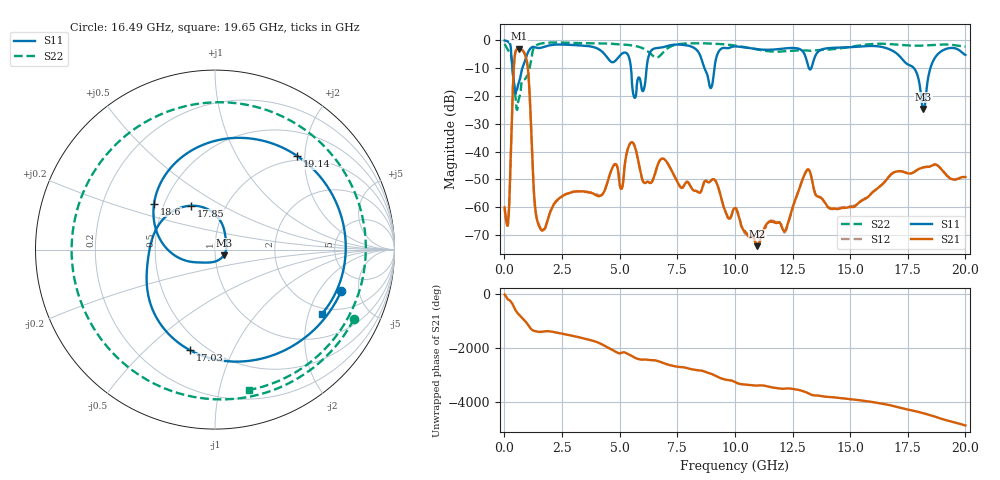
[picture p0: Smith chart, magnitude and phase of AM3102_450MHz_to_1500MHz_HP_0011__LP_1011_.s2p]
!Agilent Technologies,E8364B,MY43040894,A.07.50.67
!Agilent E8364B: A.07.50.67
!Date: Thursday, January 11, 2018 05:33:03
!Correction: S11(Full 2 Port(1,2))
!S21(Full 2 Port(1,2))
!S12(Full 2 Port(1,2))
!S22(Full 2 Port(1,2))
!S2P File: Measurements: S11, S21, S12, S22:
# Hz S  dB  R 50
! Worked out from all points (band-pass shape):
!   1601 points, 10 MHz to 20 GHz, reference 50 ohm
!   highest |S21| = -3.02 dB at 622.2 MHz (marker M1); lowest = -74.0 dB at 10.98 GHz (marker M2)
!   |S21| within 3 dB of the highest: 445.7 MHz to 929.8 MHz (484.1 MHz wide, 70.4 % of centre)
!   lowest |S11| = -24.7 dB at 18.18 GHz (marker M3), VSWR 1.12, Z = 55.1 - j3.4 ohm
!   |S11| at or under -10 dB: 5.492 GHz to 6.169 GHz (676.9 MHz wide, 11.6 % of centre); 8.68 GHz to 9.112 GHz (431.9 MHz wide, 4.86 % of centre); 17.77 GHz to 18.48 GHz (714.4 MHz wide, 3.94 % of centre)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
!   |S22| runs from -25.0 to -0.8 dB; largest |S21 - S12| = 0.0065
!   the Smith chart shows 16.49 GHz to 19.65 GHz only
!   S11 on the Smith chart (normalised r, x): 16.49 GHz: 3.21, -3.27; 17.03 GHz: 0.41, -0.69; 17.85 GHz: 0.69, +0.36; 18.6 GHz: 0.44, +0.28; 19.14 GHz: 0.91, +1.84; 19.65 GHz: 1.76, -2.44
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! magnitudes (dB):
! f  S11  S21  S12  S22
! 10 MHz  -0.1  -60.1  -60.4  -1.3
! 172.4 MHz  -0.6  -64.2  -64.4  -3.7
! 422.3 MHz  -15.5  -8.2  -8.2  -16.5
! 622.2 MHz  -15.4  -3.0  -3.0  -21.2
! 997 MHz  -4.9  -8.6  -8.6  -12.7
! 1.509 GHz  -2.8  -67.0  -66.3  -1.3
! 3.346 GHz  -1.9  -54.3  -54.4  -1.0
! 5.645 GHz  -20.6  -37.9  -37.9  -2.0
! 6.682 GHz  -2.7  -44.2  -44.1  -6.0
! 8.956 GHz  -17.2  -50.5  -50.5  -1.2
! 10.01 GHz  -2.2  -60.4  -60.2  -1.9
! 10.98 GHz  -3.2  -74.0  -73.0  -3.3
! 13.34 GHz  -9.4  -50.0  -50.0  -3.7
! 16.49 GHz  -2.6  -51.0  -51.0  -1.3
! 16.68 GHz  -3.1  -49.1  -49.1  -1.3
! 17.03 GHz  -4.8  -47.1  -47.2  -1.6
! 17.85 GHz  -11.1  -46.9  -46.9  -2.0
! 18.18 GHz  -24.7  -45.7  -45.7  -1.9
! 18.6 GHz  -7.4  -44.8  -44.8  -1.7
! 19.14 GHz  -3.2  -48.1  -48.1  -1.5
! 19.65 GHz  -3.2  -49.8  -49.9  -1.9
! 20 GHz  -5.2  -49.2  -49.3  -2.3
